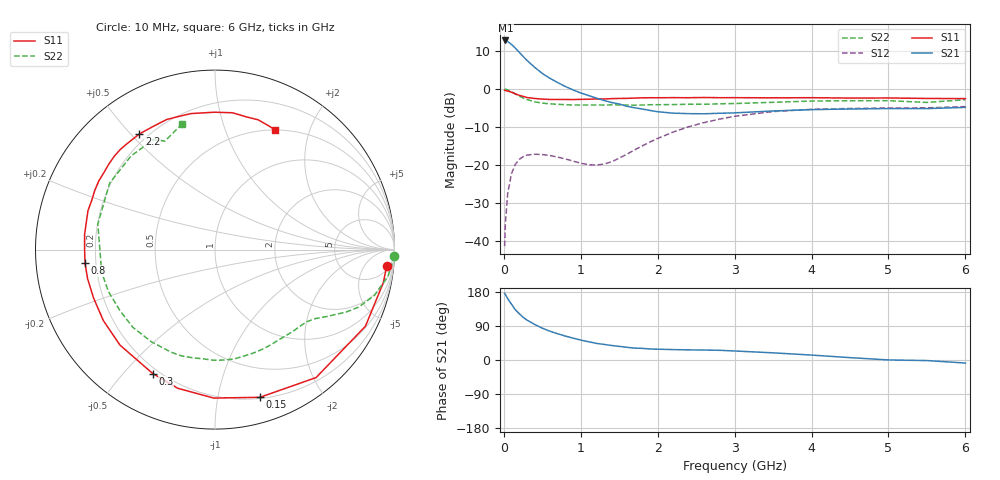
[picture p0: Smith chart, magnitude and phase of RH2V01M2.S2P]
! SIEMENS Small Signal Semiconductors
! BFR106
! Si NPN RF Bipolar Junction Transistor in SOT23
! VCE = 2 V  IC = 1.2 mA
! Common Emitter S-Parameters:  August  1996
# GHz  S  MA  R  50
!  f  S11  S21  S12  S22
! GHz  MAG  ANG  MAG  ANG  MAG  ANG  MAG  ANG
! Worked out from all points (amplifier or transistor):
!   36 points, 10 MHz to 6 GHz, reference 50 ohm
!   highest |S21| = 12.8 dB at 20 MHz (marker M1)
!   |S21| within 3 dB of that: start of sweep to 195.6 MHz
!   unconditionally stable (mu >= 1): 839.7 MHz to end of sweep
!   at 250 MHz: K = 0.28, MSG = 13.2 dB, |S12| = -17.8 dB
!   at 1.4 GHz: K = 1.46, MAG = 3.8 dB, |S12| = -19.2 dB
!   at 6 GHz: K = 1.02, MAG = -1.0 dB, |S12| = -4.6 dB
!   S11 on the Smith chart (normalised r, x): 10 MHz: 7, -18; 150 MHz: 0.21, -1.33; 300 MHz: 0.18, -0.60; 800 MHz: 0.16, -0.05; 2.2 GHz: 0.17, +0.53; 6 GHz: 0.50, +1.51
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0.01  0.9608 -5.6  4.36 175.7  0.0085 88.1  0.9986 -1.9
0.02  0.9555 -11.2  4.364 173.0  0.017 83.5  0.9944 -3.6
0.05  0.9406 -27.0  4.22 162.0  0.0419 74.8  0.9753 -8.7
0.1  0.9086 -51.7  3.868 147.0  0.0771 61.5  0.9236 -16.1
0.15  0.8601 -73.1  3.451 132.5  0.1021 49.6  0.8624 -21.8
0.2  0.8272 -90.5  3.057 122.3  0.118 41.5  0.8089 -25.5
0.25  0.8001 -105.0  2.688 112.7  0.1285 34.4  0.7607 -28.4
0.3  0.7727 -116.7  2.386 105.6  0.1345 29.6  0.7288 -30.7
0.4  0.7506 -134.9  1.936 93.9  0.1384 22.3  0.6787 -34.5
0.5  0.737 -147.6  1.602 84.0  0.1369 17.6  0.6512 -38.0
0.6  0.7284 -158.3  1.383 75.9  0.1329 15.0  0.6378 -41.9
0.8  0.7282 -174.1  1.079 63.2  0.1199 14.5  0.6212 -50.5
1.1  0.7333 167.7  0.821 48.2  0.1008 27.1  0.6148 -64.7
1.3  0.7396 158.0  0.708 41.2  0.1027 42.8  0.6146 -74.8
1.6  0.7532 145.2  0.592 33.5  0.1384 61.3  0.6164 -90.7
2.2  0.77 123.2  0.481 27.5  0.2709 63.4  0.6239 -124.5
2.8  0.7688 105.1  0.479 25.6  0.4005 49.9  0.6382 -158.6
3.5  0.7654 90.3  0.514 18.9  0.5046 32.4  0.6682 167.7
4.5  0.7598 76.6  0.545 6.2  0.5546 11.9  0.7008 131.8
5  0.7621 71.6  0.553 0.2  0.5609 4.4  0.7022 119.1
5.5  0.7516 66.6  0.552 -1.5  0.5654 0.9  0.6657 114.8
6  0.7472 63.2  0.573 -8.0  0.5865 -6.5  0.7232 104.7
